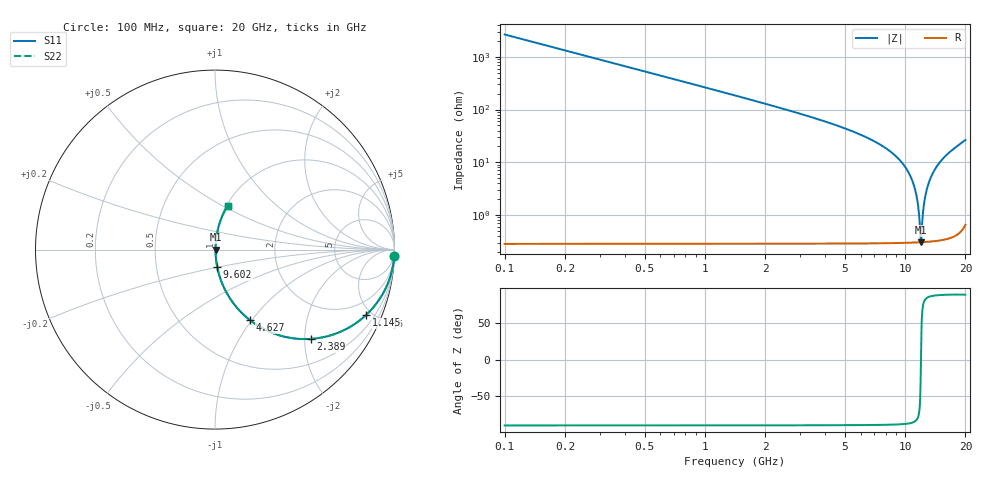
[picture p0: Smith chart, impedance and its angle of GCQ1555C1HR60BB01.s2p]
!Murata Part Number: GCQ1555C1HR60BB01
!These Parameters are Measured in Series Mode Connection
!Data Generated on Mar 13, 2026
!  o--ll--o
!Port1  Port2
!  o------o
!Operation Temp=25[degC], DC Bias Voltage=0[V]
!Freq. Start=100[MHz] Stop=20[GHz] 401[Steps]
# Hz S RI R 50
!Freq.(Hz) S11(Real) S11(Imag) S21(Real) S21(Imag) S12(Real) S12(Imag) S22(Real) S22(Imag)
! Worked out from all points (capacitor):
!   401 points, 100 MHz to 20 GHz, reference 50 ohm
!   read as one part in series: C = 600 fF near 199.5 MHz
!   lowest |Z| = 305 mohm at 11.99 GHz (marker M1)
!   series resonance near 12 GHz, so ESL is about 290 pH
!   S11 on the Smith chart (normalised r, x): 100 MHz: 1, -53; 1.145 GHz: 1.01, -4.59; 2.389 GHz: 1.01, -2.13; 4.627 GHz: 1.01, -0.98; 9.602 GHz: 1.01, -0.20; 20 GHz: 1.01, +0.53
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1e8  0.9986 -0.0376  0.00142 0.0376  0.00142 0.0376  0.9986 -0.0376
2.99e8  0.9874 -0.1114  0.0126 0.1114  0.0126 0.1114  0.9874 -0.1114
4.98e8  0.9658 -0.1816  0.0342 0.1816  0.0342 0.1816  0.9658 -0.1816
1.14475e9  0.8403 -0.3657  0.1597 0.3657  0.1597 0.3657  0.8403 -0.3657
2.3885e9  0.5323 -0.4976  0.4677 0.4976  0.4677 0.4976  0.5323 -0.4976
3.43325e9  0.3358 -0.4703  0.6642 0.4703  0.6642 0.4703  0.3358 -0.4703
4.62725e9  0.1944 -0.3928  0.8056 0.3928  0.8056 0.3928  0.1944 -0.3928
6.7665e9  0.0696 -0.2491  0.9304 0.2491  0.9304 0.2491  0.0696 -0.2491
9.60225e9  0.0128 -0.0987  0.9872 0.0987  0.9872 0.0987  0.0128 -0.0987
1.005e10  0.00919 -0.0786  0.9908 0.0786  0.9908 0.0786  0.00919 -0.0786
1.079625e10  0.00519 -0.0469  0.9948 0.0469  0.9948 0.0469  0.00519 -0.0469
1.13435e10  0.00363 -0.025  0.9964 0.025  0.9964 0.025  0.00363 -0.025
1.1642e10  0.0032 -0.0134  0.9968 0.0134  0.9968 0.0134  0.0032 -0.0134
1.199025e10  0.00303 -0.000249  0.997 0.000249  0.997 0.000249  0.00303 -0.000249
1.208975e10  0.00305 0.00345  0.997 -0.00345  0.997 -0.00345  0.00305 0.00345
1.23385e10  0.00321 0.0126  0.9968 -0.0126  0.9968 -0.0126  0.00321 0.0126
1.25375e10  0.00345 0.0197  0.9965 -0.0197  0.9965 -0.0197  0.00345 0.0197
1.288575e10  0.00412 0.0321  0.9959 -0.0321  0.9959 -0.0321  0.00412 0.0321
1.338325e10  0.00555 0.0491  0.9945 -0.0491  0.9945 -0.0491  0.00555 0.0491
1.47265e10  0.0119 0.0926  0.9881 -0.0926  0.9881 -0.0926  0.0119 0.0926
1.67165e10  0.0273 0.1516  0.9727 -0.1516  0.9727 -0.1516  0.0273 0.1516
2e10  0.0704 0.2438  0.9296 -0.2438  0.9296 -0.2438  0.0704 0.2438
